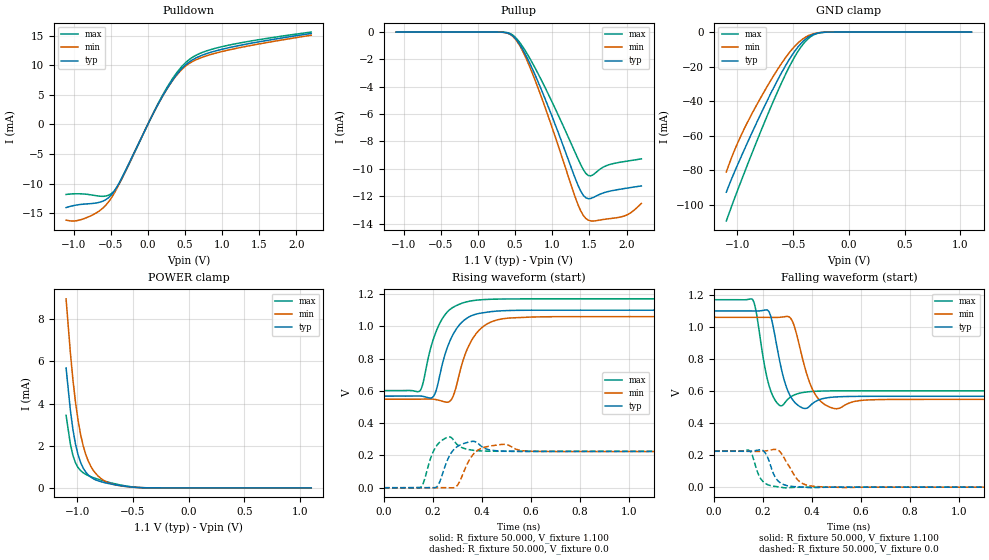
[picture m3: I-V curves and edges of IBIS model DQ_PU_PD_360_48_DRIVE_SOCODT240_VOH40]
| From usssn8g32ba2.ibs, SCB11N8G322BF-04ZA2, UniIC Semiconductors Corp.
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|   Model DQ_PU_PD_360_48_DRIVE_SOCODT240_VOH40
[Model] DQ_PU_PD_360_48_DRIVE_SOCODT240_VOH40
Model_type I/O
Polarity   Inverting
Vinl =  0.135V
Vinh =  0.305V
Vmeas =  0.220V
Rref =  50.000
Vref =  0.220V
C_comp   1.020pF   1.010pF   1.030pF
[Model Spec]
Vinh   0.305V   0.297V   0.319V
Vinl   0.135V   0.127V   0.149V
Vmeas   0.220V   0.212V   0.234V
Vref   0.220V   0.212V   0.234V
Rref   50.000   NA   NA
[Temperature Range]   25.000   0.105k   -40.000
[Voltage Range]   1.100V   1.060V   1.170V
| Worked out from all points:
|   slope of the pulldown table from 0 to 0.165 V, typ, clamps not added: 41 ohm
|   GND clamp passes 1 mA (typ) near -0.30 V on its own axis
|   POWER clamp passes 1 mA (typ) near -0.95 V on its own axis
|   rising waveform, R_fixture 50.000, V_fixture 1.100: 20-80 % time 75.3ps typ, 78.8ps min, 73.2ps max; typ from 0.567 V to 1.1 V
|   rising waveform, R_fixture 50.000, V_fixture 0.0: 20-80 % time 31.9ps typ, 40.2ps min, 25.7ps max; typ from 0 V to 0.225 V
|   falling waveform, R_fixture 50.000, V_fixture 1.100: 20-80 % time 42.9ps typ, 54.6ps min, 35.5ps max; typ from 1.1 V to 0.567 V
|   falling waveform, R_fixture 50.000, V_fixture 0.0: 20-80 % time 37.3ps typ, 55ps min, 34.4ps max; typ from 0.225 V to 0 V
[Pulldown]
|Voltage   I(typ)   I(min)   I(max)
-1.1V     -14.07mA   -16.18mA   -11.85mA
-930mV    -13.58mA   -16.22mA   -11.73mA
-726mV    -13.35mA   -15.21mA   -12mA
-556mV    -12.65mA   -13.54mA   -12.1mA
-454mV    -11.34mA   -11.69mA   -11.29mA
-318mV    -8.242mA   -8.339mA   -8.422mA
192mV     4.628mA    4.609mA    4.791mA
362mV     7.992mA    7.909mA    8.275mA
532mV     10.32mA    10.1mA     10.72mA
702mV     11.57mA    11.22mA    12.02mA
1.008V    12.75mA    12.37mA    13.19mA
2.2V      15.4mA     15.1mA     15.64mA
[Pullup]
|Voltage   I(typ)   I(min)   I(max)
-1.1V     900pA      9.618nA    0A
432mV     -147.1uA   -170.1uA   -107.3uA
568mV     -948.7uA   -1.043mA   -800.9uA
704mV     -2.351mA   -2.626mA   -1.98mA
942mV     -5.394mA   -6.093mA   -4.481mA
1.316V    -10.78mA   -12.17mA   -8.894mA
1.418V    -11.93mA   -13.4mA    -10.05mA
1.52V     -12.16mA   -13.81mA   -10.51mA
1.724V    -11.7mA    -13.67mA   -9.778mA
1.928V    -11.48mA   -13.51mA   -9.507mA
2.064V    -11.36mA   -13.18mA   -9.389mA
2.2V      -11.25mA   -12.53mA   -9.27mA
[GND_clamp]
|Voltage   I(typ)   I(min)   I(max)
-1.1V     -92.78mA   -81.05mA   -109.5mA
-1.031V   -81.73mA   -69.22mA   -97.17mA
-939mV    -68.18mA   -56.02mA   -81.64mA
-824mV    -52mA      -41.83mA   -62.83mA
-686mV    -33.62mA   -26.41mA   -41.32mA
-571mV    -19.76mA   -15.06mA   -24.85mA
-479mV    -10.5mA    -7.76mA    -13.5mA
-410mV    -5.313mA   -3.84mA    -6.916mA
-341mV    -2.007mA   -1.45mA    -2.59mA
-272mV    -506.9uA   -403.5uA   -609.8uA
-180mV    -45.65uA   -51.35uA   -43.55uA
1.1V      0A         0A         0A
[POWER_clamp]
|Voltage   I(typ)   I(min)   I(max)
-1.1V     5.691mA    8.967mA    3.44mA
-1.062V   3.709mA    6.444mA    2.092mA
-1.039V   2.781mA    5.152mA    1.546mA
-1.016V   2.086mA    4.085mA    1.193mA
-970mV    1.21mA     2.539mA    818.5uA
-947mV    943.7uA    2.005mA    716.7uA
-901mV    610.1uA    1.27mA     581.3uA
-855mV    430.7uA    824.1uA    484.6uA
-786mV    289.9uA    439.4uA    366uA
-671mV    155.9uA    155.9uA    203.6uA
-441mV    13.2uA     12.79uA    15.03uA
1.1V      0A         0A         0A
[Ramp]
| variable   typ   min   max
dV/dt_r   0.135/31.898p   0.134/40.354p   0.135/25.738p
dV/dt_f   0.320/43.098p   0.307/54.690p   0.341/35.586p
R_load = 50.000
[Rising Waveform]
R_fixture= 50.000
V_fixture= 1.100
V_fixture_min= 1.060
V_fixture_max= 1.170
|time   V(typ)   V(min)   V(max)
0s        567.3mV    548.1mV    601.6mV
147ps     568.1mV    548.7mV    600.9mV
207ps     578.8mV    547.3mV    944.5mV
268ps     905.3mV    534.8mV    1.103V
288ps     965.8mV    590.9mV    1.123V
333ps     1.045V     833.5mV    1.15V
370ps     1.073V     942.3mV    1.161V
442ps     1.092V     1.03V      1.168V
592ps     1.1V       1.057V     1.17V
3ns       1.1V       1.06V      1.17V
[Rising Waveform]
R_fixture= 50.000
V_fixture= 0.0
V_fixture_min= 0.0
V_fixture_max= 0.0
|time   V(typ)   V(min)   V(max)
0s        2.854uV    10.37uV    664nV
151ps     134.1uV    28.38uV    3.872mV
195ps     275.2uV    124.4uV    201.8mV
217ps     7.6mV      347.7uV    264.6mV
264ps     188.1mV    -29.45uV   314.9mV
299ps     254.8mV    13.91mV    267mV
373ps     285mV      220.8mV    230.5mV
482ps     227.1mV    268.3mV    225.7mV
605ps     224.8mV    225.6mV    225.5mV
3ns       224.7mV    224.1mV    225.5mV
[Falling Waveform]
R_fixture= 50.000
V_fixture= 1.100
V_fixture_min= 1.060
V_fixture_max= 1.170
|time   V(typ)   V(min)   V(max)
0s        1.1V       1.06V      1.17V
158ps     1.1V       1.06V      1.169V
225ps     1.093V     1.06V      632.3mV
271ps     766.1mV    1.061V     508.5mV
313ps     565.1mV    1.054V     563.4mV
351ps     502.7mV    868.7mV    587.2mV
410ps     530.8mV    587.7mV    598.2mV
493ps     562.8mV    490.5mV    601.1mV
692ps     567.3mV    547.2mV    601.6mV
3ns       567.3mV    548.1mV    601.6mV
[Falling Waveform]
R_fixture= 50.000
V_fixture= 0.0
V_fixture_min= 0.0
V_fixture_max= 0.0
|time   V(typ)   V(min)   V(max)
0s        224.7mV    224.1mV    225.5mV
143ps     224.3mV    223.8mV    229.2mV
182ps     232.3mV    223.4mV    77.45mV
198ps     230.6mV    224.3mV    38.84mV
217ps     192.6mV    227.6mV    17.2mV
254ps     52.75mV    235.4mV    3.868mV
292ps     12.46mV    167.1mV    -4.066mV
348ps     1.967mV    36.79mV    -501.6uV
436ps     -1.092mV   2.501mV    -14.69uV
3ns       -1.696uV   10.25uV    521nV
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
